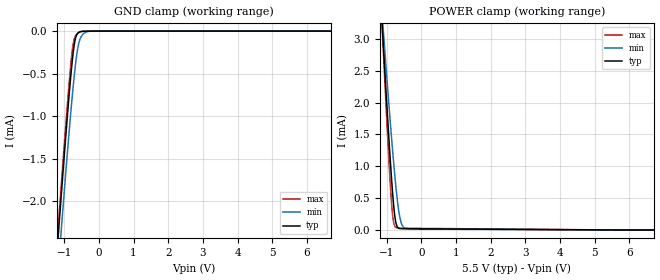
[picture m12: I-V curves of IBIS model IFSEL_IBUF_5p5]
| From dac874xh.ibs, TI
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|   IFSEL_IBUF_5p5 Model
[Model]   IFSEL_IBUF_5p5
Model_type   Input
Vinl = 1.65
Vinh = 3.85
|   typ   min   max
C_comp   1.62855E-13  6.2518E-14   2.17306E-13
| Where nom  PVT is Nominal Process, 5.5V, 27C
|   Fast PVT is Strong Process,  5.501V, -40C
|   Slow PVT is Weak Process,   5.499V, 150C
[Model spec]
|subparameter
Vinl   1.65   1.6497   1.6503
Vinh   3.85   3.8493   3.8507
[Voltage Range]   5.5   5.499   5.501
[Temperature Range]   27   150   -40
[Power Clamp Reference]   5.5   5.499   5.501
[GND Clamp Reference]   0   0   0
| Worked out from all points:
|   GND clamp passes 1 mA (typ) near -0.91 V on its own axis
|   POWER clamp passes 1 mA (typ) near -0.88 V on its own axis
[GND Clamp]
|   Voltage   I(typ)   I(min)   I(max)
-5.5V     -27.55mA   -27.35mA   -28.01mA
-1.359V   -3.459mA   -3.825mA   -3.368mA
-1.177V   -2.446mA   -2.842mA   -2.336mA
-1.161V   -2.355mA   -2.754mA   -2.243mA
-1.127V   -2.173mA   -2.578mA   -2.058mA
-1.028V   -1.637mA   -2.057mA   -1.511mA
-880mV    -867.2uA   -1.302mA   -726.9uA
-781mV    -411.6uA   -834uA     -280.2uA
-682mV    -100uA     -426.7uA   -64.77uA
-550mV    -9.064uA   -103.4uA   -12.3uA
-220mV    -713.4nA   -789.4nA   -972.6nA
11V       0A         0A         0A
[POWER Clamp]
|   Voltage   I(typ)   I(min)   I(max)
-5.5V     48.93mA    43.07mA    56.41mA
-1.127V   3.21mA     3.369mA    3.176mA
-1.095V   2.895mA    3.125mA    2.802mA
-929.5mV  1.385mA    1.935mA    1.038mA
-847mV    716.2uA    1.374mA    342uA
-814mV    486.5uA    1.16mA     167.8uA
-764.5mV  218.3uA    856.1uA    58.64uA
-698.5mV  53.93uA    500.1uA    33.23uA
-632.5mV  24.1uA     235.1uA    28.59uA
-550mV    20.37uA    71.82uA    27.31uA
-286mV    19.26uA    14.3uA     26.04uA
11V       0A         0A         0A
